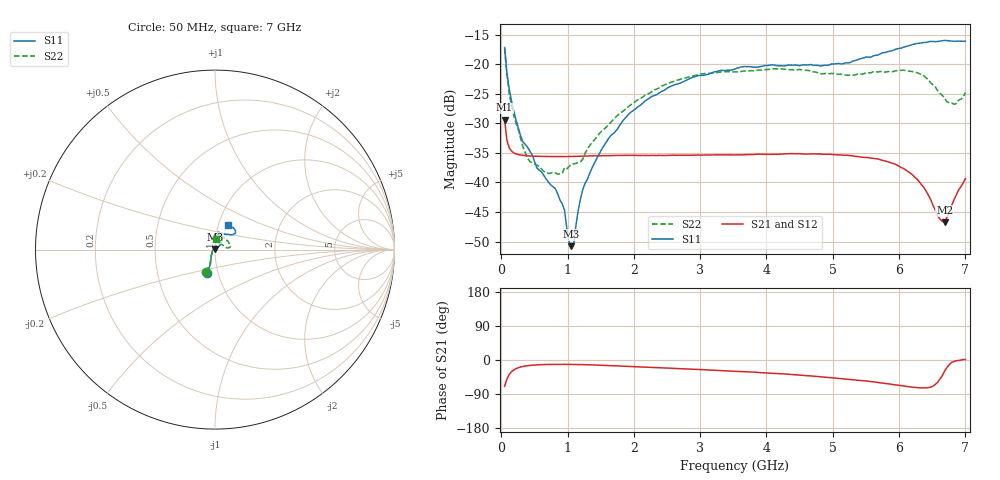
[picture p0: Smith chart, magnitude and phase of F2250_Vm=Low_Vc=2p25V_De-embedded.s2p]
! Integrated Device Technology
! Corporate Headquarters
! 6024 Silver Creek Valley Road
! San Jose, CA 95138  USA
! Phone:  1-408-284-8200
! Toll Free:  1-800-223-1366
! Webpage:  http://www.idt.com/
! Timing and RF Division
! 515 Groton Road, Suite 102
! Westford, MA 01886-6024
! Device:  F2250
! Description: Voltage Variable RF Attenuator
! Frequency:  50.0 -  6000.00 MHz
! Package:  3x3 mm Thin QFN Plastic Package: 16 pin
! Ports:  2 RF, 3 DC
!  Pin  1  = GND
!  Pin  2  = NC
!  Pin  3  = RF1  = Port 1
!  Pin  4  = NC
!  Pin  5  = GND
!  Pin  6  = GND
!  Pin  7  = GND
!  Pin  8  = GND
!  Pin  9  = NC
!  Pin 10  = RF2  = Port 2
!  Pin 11  = NC
!  Pin 12  = GND
!  Pin 13  = GND
!  Pin 14  = VCNTRL
!  Pin 15  = VDD
!  Pin 16  = VMODE
! Vcntrl:  2.250 Volts
! Vmode:  +0.000 Volts
! Vdd:  +3.30  Volts
! Current:  1.177 mA
! Data:  The device was measured on a the F2250 evaluation board which has
!  individual transmission lines to the RF pins.  Data was collected
!  using a calibrated network analyzer.  The evaluation board was
!  de-embedded using a TRL calibration technique.
!  The reference plane is the edge of the package pin.
! Misc:  SN 10
!  Action Tracker AT0258
! Date Measured:  2014-11-26
! Date:  2015-10-15  MJV
! Note:
!  Integrated Device Technology supplies this data as a sample of measured
!  data at the package pin for this product.  Your particular data for this
!  product may vary.
!  Data was taken at 25 degrees C.
!  Integrated Device Technology reserves the right to change this data at anytime.
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# GHz S dB R 50
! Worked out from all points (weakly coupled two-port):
!   201 points, 50 MHz to 7 GHz, reference 50 ohm
!   highest |S21| = -29.39 dB at 50 MHz (marker M1); lowest = -46.7 dB at 6.687 GHz (marker M2)
!   lowest |S11| = -50.8 dB at 1.058 GHz (marker M3), VSWR 1.01, Z = 49.8 + j0.243 ohm
!   |S11| at or under -10 dB: start of sweep to end of sweep
!   |S22| runs from -38.6 to -17.4 dB; largest |S21 - S12| = 7e-05
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0.05  -17.18 -108.6  -29.39 -69.6  -29.39 -69.6  -17.36 -110.6
0.08475  -21.44 -107.4  -32.88 -50.2  -32.88 -50.1  -21.87 -109.3
0.15425  -26.23 -116.6  -34.70 -31.0  -34.70 -31.0  -27.03 -120.7
0.29325  -32.20 -127.8  -35.37 -18.4  -35.37 -18.4  -32.56 -134.6
0.3975  -34.09 -141.7  -35.50 -14.9  -35.50 -15.0  -35.89 -158.1
0.6755  -39.40 -163.6  -35.61 -11.9  -35.60 -11.9  -38.31 158.1
0.91875  -43.60 158.3  -35.62 -11.5  -35.62 -11.5  -38.50 129.0
0.9535  -44.69 169.6  -35.62 -11.5  -35.62 -11.6  -37.52 126.9
1.023  -50.05 144.4  -35.61 -11.6  -35.61 -11.6  -37.28 110.5
1.05775  -50.77 122.6  -35.61 -11.7  -35.61 -11.6  -36.89 105.2
1.0925  -50.40 90.6  -35.59 -11.8  -35.60 -11.7  -36.84 100.3
1.162  -44.62 56.7  -35.57 -11.9  -35.58 -11.9  -36.61 89.4
1.2315  -41.11 44.4  -35.55 -12.2  -35.55 -12.1  -36.00 79.8
1.6485  -32.11 41.9  -35.47 -14.7  -35.46 -14.7  -29.88 61.5
2.37825  -24.87 47.3  -35.42 -20.4  -35.42 -20.4  -24.02 55.3
3.525  -20.80 72.5  -35.35 -29.6  -35.35 -29.6  -21.32 74.1
4.7065  -20.17 72.4  -35.16 -42.7  -35.15 -42.7  -21.30 71.8
5.85325  -17.82 40.5  -36.58 -63.4  -36.58 -63.4  -21.23 22.2
6.27025  -16.51 40.1  -39.42 -72.6  -39.43 -72.7  -21.44 8.8
6.68725  -15.99 48.8  -46.72 -28.9  -46.70 -28.4  -25.82 27.7
6.861  -16.12 55.1  -42.16 -2.0  -42.12 -2.1  -26.68 57.9
7  -16.12 63.3  -39.35 1.2  -39.29 1.1  -24.78 83.6
